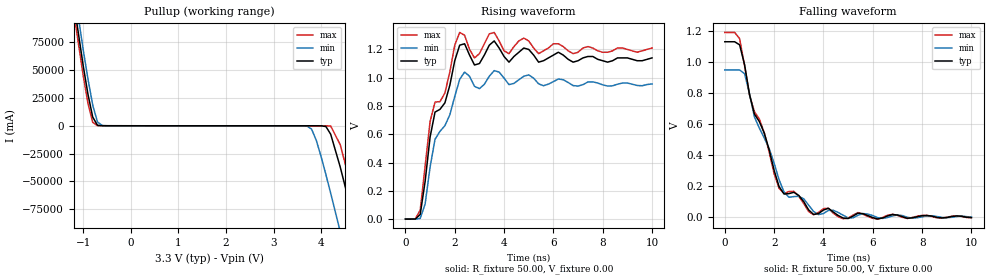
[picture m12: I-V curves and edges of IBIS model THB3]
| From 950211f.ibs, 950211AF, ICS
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|   Model THB3
[Model]   THB3
Model_type   Open_source
Polarity   Non-Inverting
|Vinl = 800.00mV
|Vinh =   2.00V
C_comp   5.50pF   5.00pF   6.00pF
[Temperature Range]   27.00   70.00   0.00
[Voltage Range]   3.30V   3.00V   3.40V
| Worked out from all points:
|   slope of the pullup table from 0 to 0.495 V, typ, clamps not added: 43.6 ohm
|   rising waveform, R_fixture 50.00, V_fixture 0.00: 20-80 % time 979ps typ, 978ps min, 989ps max; typ from 0 V to 1.14 V
|   falling waveform, R_fixture 50.00, V_fixture 0.00: 20-80 % time 1.27ns typ, 1.28ns min, 1.27ns max; typ from 1.13 V to -0.005 V
[Pullup]
| voltage   I(typ)   I(min)   I(max)
-3.3V     742.7A     756.1A     734.5A
-1.5V     197.8A     212.2A     188.9A
-1V       53.97A     68.3A      45.07A
-800mV    7.78A      18.54A     3.05A
-700mV    435.9mA    3.38A      88.47mA
3.7V      -23.03mA   -201.2mA   -24.36mA
3.9V      -24.01mA   -13.45A    -24.43mA
4.2V      -7.59A     -60.64A    -198mA
4.4V      -36.96A    -95.14A    -17A
4.6V      -70.81A    -130.3A    -49.32A
4.8V      -105.8A    -166A      -83.96A
6.2V      -358.7A    -419.6A    -336.6A
[Ramp]
| variable   typ   min   max
dV/dt_r   682.80m/928.74p   573.60m/939.16p   723.60m/924.18p
dV/dt_f   679.04m/1.20   570.08m/1.20n   719.67m/1.20n
[Rising Waveform]
R_fixture = 50.00
V_fixture = 0.00
V_fixture_min = 0.00
V_fixture_max = 0.00
| time   V(typ)   V(min)   V(max)
0s        0V         0V         0V
600ps     32.62mV    4.34mV     64.08mV
1ns       580.4mV    367.3mV    689.5mV
1.6ns     821.7mV    660.4mV    891.7mV
2.2ns     1.23V      988mV      1.32V
2.8ns     1.09V      939mV      1.14V
3.6ns     1.26V      1.05V      1.32V
4.2ns     1.11V      951.1mV    1.17V
4.8ns     1.21V      1.01V      1.28V
10ns      1.14V      956mV      1.21V
[Falling Waveform]
R_fixture = 50.00
V_fixture = 0.00
V_fixture_min = 0.00
V_fixture_max = 0.00
| time   V(typ)   V(min)   V(max)
0s        1.13V      948.5mV    1.19V
600ps     1.11V      948mV      1.15V
800ps     982.7mV    923.9mV    974.7mV
1.2ns     663.1mV    645.2mV    678.8mV
1.6ns     540mV      509mV      542mV
2.2ns     195.3mV    239.4mV    183.8mV
2.4ns     147.4mV    160.1mV    150.9mV
2.8ns     158.4mV    130.6mV    164.6mV
3.8ns     20.95mV    14.53mV    28.89mV
10ns      -4.72mV    -1.63mV    -5.45mV
